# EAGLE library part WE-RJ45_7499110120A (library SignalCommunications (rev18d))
WE-RJ45 LAN Transformer Order Code 7499110120A Design THT xBase-T 10/100/1000 Base-T Ports 1x1 Application Standard Tab Position Vertical LED (Left-Right) YELLOW-GREEN EMI Fingers No Details see: http://katalog.we-online.de/en/pbs/WE-LAN-RJ45 Created by Yingchun Shan 2016 (C) Wurth Elektronik
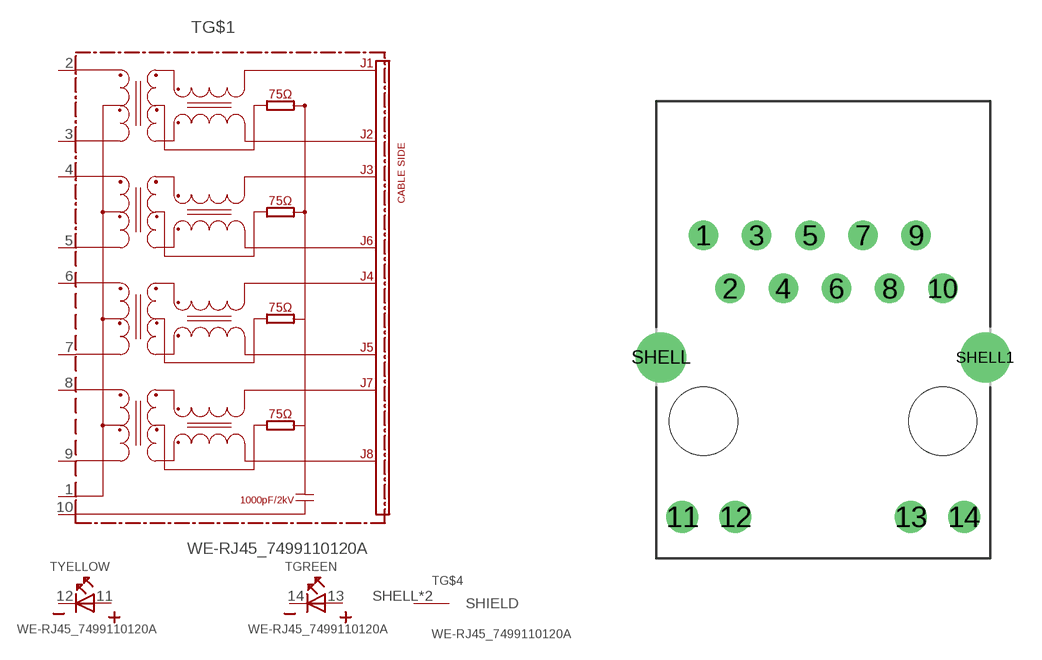
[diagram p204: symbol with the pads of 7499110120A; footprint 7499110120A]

Designator prefix T; gates G$1=7499110120A YELLOW=LED_2PIN GREEN=LED_2PIN G$4=SHIELD

## WE-RJ45_7499110120A  [7499110120A]
1  G$1:1
2  G$1:2
3  G$1:3
4  G$1:4
5  G$1:5
6  G$1:6
7  G$1:7
8  G$1:8
9  G$1:9
10  G$1:10
11  YELLOW:A  pas
12  YELLOW:K  pas
13  GREEN:A  pas
14  GREEN:K  pas
SHELL  G$4:SHIELD  pas
SHELL1  G$4:SHIELD  pas

## Footprint 7499110120A (pad centres in mm)
drill 0.9: 1 -5.715,8.89; 2 -4.445,6.35; 3 -3.175,8.89; 4 -1.905,6.35; 5 -0.635,8.89; 6 0.635,6.35; 7 1.905,8.89; 8 3.175,6.35; 9 4.445,8.89; 10 5.715,6.35
drill 1.02: 11 -6.73,-4.57; 12 -4.19,-4.57; 13 4.19,-4.57; 14 6.73,-4.57
drill 1.6: SHELL -7.745,3.05; SHELL1 7.745,3.05
hole 3.25 at -5.715,0
hole 3.25 at 5.715,0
